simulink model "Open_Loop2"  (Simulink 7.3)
settings: Solver=ode45  StartTime=0.0  StopTime=10.0  RelTol=1e-3
undefined symbols (not defined in the file or in its folder): Aol, Bol, Col, Dol

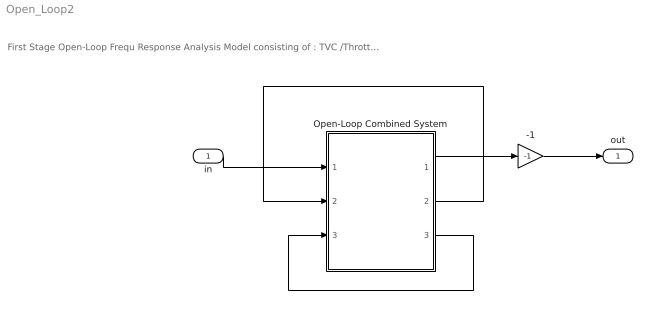
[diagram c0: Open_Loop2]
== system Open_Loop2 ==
  note: First Stage Open-Loop Frequ Response Analysis Model consisting of : TVC /Throttle Control, Flight Control, Vehicle and Actuators Combined using Flixan (Open-Loop System)
  in : Inport  OutDataType=sfix(16)  OutScaling=2^0
  -1 : Gain  Gain=-1  ParameterDataType=sfix(16)  ParameterScaling=2^0  OutDataType=sfix(16)  OutScaling=2^0
  Open-Loop Combined System : Subsystem
  out : Outport  OutDataType=sfix(16)  OutScaling=2^0
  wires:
  -1/1 -> out/1
  Open-Loop Combined System/2(Dq_Tvc) -> Open-Loop Combined System/2(DQ-TVC)
  in/1 -> Open-Loop Combined System/1(DP-TVC)
  Open-Loop Combined System/1(Dp_Tvc) -> -1/1
  Open-Loop Combined System/3(Dr_Tvc) -> Open-Loop Combined System/3(DR-TVC)

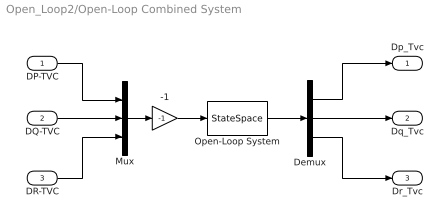
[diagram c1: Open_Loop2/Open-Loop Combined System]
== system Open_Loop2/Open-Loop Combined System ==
  DP-TVC : Inport  OutDataType=sfix(16)  OutScaling=2^0
  DQ-TVC : Inport  Port=2  OutDataType=sfix(16)  OutScaling=2^0
  DR-TVC : Inport  Port=3  OutDataType=sfix(16)  OutScaling=2^0
  -1 : Gain  Gain=-1  ParameterDataType=sfix(16)  ParameterScaling=2^0  OutDataType=sfix(16)  OutScaling=2^0
  Demux : Demux  Outputs=3
  Mux : Mux  Inputs=3
  Open-Loop System : StateSpace  A=Aol  B=Bol  C=Col  D=Dol
  Dp_Tvc : Outport  OutDataType=sfix(16)  OutScaling=2^0
  Dq_Tvc : Outport  Port=2  OutDataType=sfix(16)  OutScaling=2^0
  Dr_Tvc : Outport  Port=3  OutDataType=sfix(16)  OutScaling=2^0
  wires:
  Open-Loop System/1 -> Demux/1
  Mux/1 -> -1/1
  DP-TVC/1 -> Mux/1
  DQ-TVC/1 -> Mux/2
  DR-TVC/1 -> Mux/3
  Demux/1 -> Dp_Tvc/1
  Demux/2 -> Dq_Tvc/1
  Demux/3 -> Dr_Tvc/1
  -1/1 -> Open-Loop System/1
